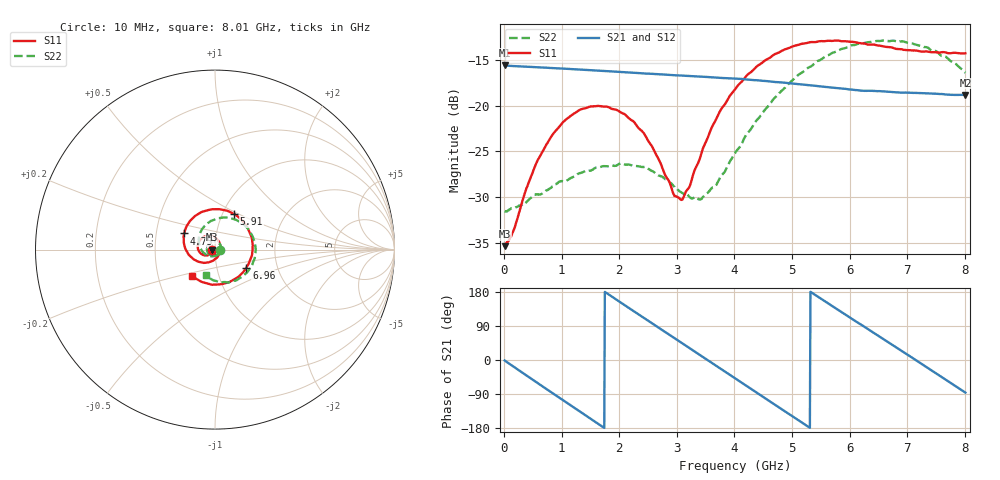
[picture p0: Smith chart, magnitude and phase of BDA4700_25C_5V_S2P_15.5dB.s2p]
!Agilent Technologies,E5071B,MY42404982,A.09.10
!Date: Mon Oct 20 13:33:59 2025
!Data & Calibration Information:
!Freq	S11:SOLT2(ON)	S21:SOLT2(ON)	S12:SOLT2(ON)	S22:SOLT2(ON)
# Hz S RI R 50
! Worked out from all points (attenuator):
!   801 points, 10 MHz to 8.01 GHz, reference 50 ohm
!   highest |S21| = -15.60 dB at 10 MHz (marker M1); lowest = -18.8 dB at 8.01 GHz (marker M2)
!   lowest |S11| = -35.3 dB at 10 MHz (marker M3), VSWR 1.03, Z = 48.3 - j0.108 ohm
!   |S11| at or under -10 dB: start of sweep to end of sweep
!   |S22| runs from -31.6 to -12.9 dB; largest |S21 - S12| = 0.0012
!   S11 on the Smith chart (normalised r, x): 10 MHz: 0.97, -0.00; 4.75 GHz: 0.70, +0.13; 5.91 GHz: 1.13, +0.47; 6.96 GHz: 1.39, -0.29; 8.01 GHz: 0.75, -0.23
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1e7  -0.0171 -0.00112  0.1659 -0.00358  0.1658 -0.00383  0.0265 -0.00103
1.5e8  -0.0181 -0.00924  0.1582 -0.0452  0.1582 -0.0453  0.0265 -0.0076
4.1e8  -0.0272 -0.0247  0.1194 -0.1111  0.1194 -0.1112  0.02 -0.0226
7e8  -0.0485 -0.0328  0.0476 -0.1542  0.0476 -0.1541  0.00421 -0.0336
1.03e9  -0.0784 -0.0224  -0.0458 -0.1526  -0.0459 -0.1526  -0.0203 -0.0328
1.35e9  -0.0956 0.00679  -0.1195 -0.1022  -0.1195 -0.1023  -0.0406 -0.0144
1.72e9  -0.0857 0.0494  -0.1546 -0.00748  -0.1547 -0.0075  -0.0436 0.0169
2.09e9  -0.0485 0.0757  -0.1251 0.0869  -0.1252 0.0869  -0.0234 0.0417
2.42e9  -0.00541 0.0711  -0.0559 0.1391  -0.056 0.1392  0.00574 0.0459
2.68e9  0.0209 0.0468  0.011 0.1481  0.011 0.1481  0.0241 0.0339
2.95e9  0.0311 0.00958  0.0765 0.1252  0.0764 0.125  0.0334 0.0139
3.1e9  0.028 -0.0128  0.1059 0.1003  0.1056 0.1006  0.0333 -7.46e-05
3.43e9  -0.00257 -0.0554  0.1417 0.026  0.1417 0.0259  0.0165 -0.0262
3.75e9  -0.0571 -0.0737  0.1318 -0.0524  0.1319 -0.0526  -0.0152 -0.0376
4.01e9  -0.1065 -0.0607  0.0941 -0.1044  0.0942 -0.1043  -0.0457 -0.0305
4.75e9  -0.1719 0.0898  -0.0725 -0.1131  -0.0723 -0.1134  -0.0889 0.0719
5.35e9  -0.0644 0.2127  -0.1287 0.00671  -0.1287 0.0064  -0.00685 0.1654
5.91e9  0.1051 0.199  -0.0641 0.1057  -0.0644 0.1055  0.1318 0.158
6.68e9  0.2082 -0.0159  0.0829 0.0854  0.0832 0.0853  0.2241 -0.0248
6.96e9  0.1746 -0.1009  0.1117 0.0375  0.1117 0.037  0.1991 -0.0997
7.49e9  0.03 -0.1935  0.0961 -0.0653  0.096 -0.0654  0.0772 -0.1834
8.01e9  -0.126 -0.1466  0.00797 -0.114  0.00806 -0.1141  -0.0512 -0.1422
